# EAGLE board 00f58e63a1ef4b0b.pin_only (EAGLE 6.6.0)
REV: B

Size 55.88 x 22.86 mm. Coordinates in mm from the lower left corner, seen from the top.
Outline: 0,20.32 0,2.54 arc90 2.54,0 53.34,0 arc90 55.88,2.54 55.88,20.32 arc90 53.34,22.86 2.54,22.86 arc90 0,20.32
Copper layers (1*16): Top 0.035mm / dielectric 1.5mm / Bottom 0.035mm
Design rules "adafruit *": minimum track width 8mil, minimum drill 15.5mil, track to track 8mil, track to pad 8mil, pad to pad 8mil, via to via 8mil, smd to smd 8mil, copper to edge 10mil, drill to drill 8mil, minimum pad ring 10mil, minimum via ring 8mil, stop-mask expansion 2mil, vias tented up to drill 20mil, thermal gap 10mil

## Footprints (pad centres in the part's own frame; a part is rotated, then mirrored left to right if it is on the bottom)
0603-NO = smd 1.1 x 1: 1 -0.85,0; 2 0.85,0
0805-NO = smd 1.24 x 1.5: 1 -0.95,0; 2 0.95,0
FIDUCIAL_1MM = smd 1 x 1: 1 0,0
SOT23-5L = smd 0.55 x 1.2: 1 -0.95,-1.3; 2 0,-1.3; 3 0.95,-1.3; 4 0.95,1.3; 5 -0.95,1.3
1X03_ROUND_76 = drill 1 pad 1.93: 1 -2.54,0; 2 0,0; 3 2.54,0
1X13_ROUND_70 = drill 1 pad 1.676: 1 -15.24,0; 2 -12.7,0; 3 -10.16,0; 4 -7.62,0; 5 -5.08,0; 6 -2.54,0; 7 0,0; 8 2.54,0; 9 5.08,0; 10 7.62,0; 11 10.16,0; 12 12.7,0; 13 15.24,0
1X09_ROUND_70 = drill 1 pad 1.778: 1 -10.16,0; 2 -7.62,0; 3 -5.08,0; 4 -2.54,0; 5 0,0; 6 2.54,0; 7 5.08,0; 8 7.62,0; 9 10.16,0
FEATHERWING_NODIM = drill 1 pad 1.778: 1 6.35,1.27; 2 8.89,1.27; 3 11.43,1.27; 4 13.97,1.27; 5 16.51,1.27; 6 19.05,1.27; 7 21.59,1.27; 8 24.13,1.27; 9 26.67,1.27; 10 29.21,1.27; 11 31.75,1.27; 12 34.29,1.27; 13 36.83,1.27; 14 39.37,1.27; 15 41.91,1.27; 16 44.45,1.27; 17 44.45,21.59; 18 41.91,21.59; 19 39.37,21.59; 20 36.83,21.59; 21 34.29,21.59; 22 31.75,21.59; 23 29.21,21.59; 24 26.67,21.59; 25 24.13,21.59; 26 21.59,21.59; 27 19.05,21.59; 28 16.51,21.59 | drill 2.5 pad 3.81: P$1 2.54,20.32; P$2 2.54,2.54 | hole 2.54: 48.26,20.32; 48.26,2.54
SOLDERJUMPER_REFLOW_NOPASTE = smd 1.168 x 1.6: 1 -0.762,0; 2 0.762,0
SOLDERJUMPER_CLOSEDWIRE = smd 1.168 x 1.6: 1 -0.762,0; 2 0.762,0 | smd 0.635 x 0.203: WIRE 0,0
BTN_KMR2_4.6X2.8 = smd 0.9 x 0.9: A 2.05,0.8; A' -2.05,0.8; B 2.05,-0.8; B' -2.05,-0.8
LQFP48 = smd 1.1 x 0.285: 1 -4.2,2.75; 2 -4.2,2.25; 3 -4.2,1.75; 4 -4.2,1.25; 5 -4.2,0.75; 6 -4.2,0.25; 7 -4.2,-0.25; 8 -4.2,-0.75; 9 -4.2,-1.25; 10 -4.2,-1.75; 11 -4.2,-2.25; 12 -4.2,-2.75; 25 4.2,-2.75; 26 4.2,-2.25; 27 4.2,-1.75; 28 4.2,-1.25; 29 4.2,-0.75; 30 4.2,-0.25; 31 4.2,0.25; 32 4.2,0.75; 33 4.2,1.25; 34 4.2,1.75; 35 4.2,2.25; 36 4.2,2.75 | smd 0.285 x 1.1: 13 -2.75,-4.2; 14 -2.25,-4.2; 15 -1.75,-4.2; 16 -1.25,-4.2; 17 -0.75,-4.2; 18 -0.25,-4.2; 19 0.25,-4.2; 20 0.75,-4.2; 21 1.25,-4.2; 22 1.75,-4.2; 23 2.25,-4.2; 24 2.75,-4.2; 37 2.75,4.2; 38 2.25,4.2; 39 1.75,4.2; 40 1.25,4.2; 41 0.75,4.2; 42 0.25,4.2; 43 -0.25,4.2; 44 -0.75,4.2; 45 -1.25,4.2; 46 -1.75,4.2; 47 -2.25,4.2 | smd 0.28 x 1.1: 48 -2.75,4.2
RJ45_PULSEJACK = drill 0.9 pad 1.676: 1 4.445,-6.35; 2 3.175,-8.89; 3 1.905,-6.35; 4 0.635,-8.89; 5 -0.635,-6.35; 6 -1.905,-8.89; 7 -3.175,-6.35; 8 -4.445,-8.89 | drill 1 pad 1.676: 9 6.325,4.9; 10 3.785,3.38; 11 -3.785,4.9; 12 -6.325,3.38 | drill 1.6: P$5 -7.875,-3.05; P$6 7.875,-3.05 | hole 3.2: -5.715,0; 5.715,0
CRYSTAL_3.2X2.5 = smd 1.4 x 1.2: 1 -1.1,-0.8; 2 1.1,0.8; GND1 -1.1,0.8; GND2 1.1,-0.8

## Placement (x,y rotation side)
C1  22pF  [0603-NO]  7.62,8.64 180 top
C2  22pF  [0603-NO]  7.24,14.48 180 top
C3  6.8nF  [0603-NO]  35.56,15.88 180 top
C4  6.8nF  [0603-NO]  35.56,17.27 180 top
C5  10nF  [0603-NO]  35.56,13.08 180 top
C6  10nF  [0603-NO]  35.56,10.29 180 top
C7  0.1uF  [0603-NO]  22.73,16.13 270 top
C8  0.1uF  [0603-NO]  24.13,16.13 270 top
C9  0.1uF  [0603-NO]  25.53,16.13 270 top
C10  0.1uF  [0603-NO]  26.92,16.13 270 top
C11  10uF  [0805-NO]  28.57,16.13 270 top
C12  10uF  [0805-NO]  13.97,20.07 90 top
C13  0.1uF  [0603-NO]  12.83,16.76 180 top
C14  10uF  [0805-NO]  6.6,6.22 90 top
C15  0.1uF  [0603-NO]  8.38,6.35 90 top
FB1  ferrite  [0805-NO]  10.79,18.29 0 top
FB2  ferrite  [0805-NO]  29.08,7.87 0 top
FID1  FIDUCIAL""  [FIDUCIAL_1MM]  46.48,1.02 0 top
FID2  FIDUCIAL""  [FIDUCIAL_1MM]  1.02,5.21 0 top
FID3  FIDUCIAL""  [FIDUCIAL_1MM]  46.48,21.84 0 top
IC1  74AHC1G125  [SOT23-5L]  11.05,7.37 180 top
JP1  [1X03_ROUND_76]  2.54,11.43 270 top
JP2  [1X13_ROUND_70]  21.59,3.3 180 top
JP4  [1X09_ROUND_70]  26.67,19.43 0 top
MS1  FEATHERWING_NODIM  [FEATHERWING_NODIM]  0,0 0 top
R1  12.4K  [0603-NO]  24.51,13.59 0 top
R2  1M  [0603-NO]  10.16,11.18 90 top
R3  10K  [0603-NO]  3.94,17.14 0 top
R4  49.9  [0603-NO]  35.56,7.49 180 top
R5  10K  [0603-NO]  25.65,8.13 180 top
R6  10K  [0603-NO]  25.65,6.73 180 top
R7  10K  [0603-NO]  25.65,5.4 180 top
R8  10K  [0603-NO]  13.74,6.48 90 top
R9  49.9  [0603-NO]  35.56,6.1 180 top
R10  49.9  [0603-NO]  35.56,14.48 180 top
R11  49.9  [0603-NO]  35.56,11.68 180 top
R12  10  [0603-NO]  35.56,8.89 180 top
R13  470  [0603-NO]  53.21,20.83 180 top
R14  470  [0603-NO]  53.21,2.16 180 top
R15  10K  [0603-NO]  3.94,15.75 0 top
SJ1  [SOLDERJUMPER_REFLOW_NOPASTE]  18.29,11.68 0 bottom
SJ2  [SOLDERJUMPER_REFLOW_NOPASTE]  18.29,9.4 0 bottom
SJ3  [SOLDERJUMPER_REFLOW_NOPASTE]  18.29,7.11 180 bottom
SJ4  [SOLDERJUMPER_CLOSEDWIRE]  5.84,17.53 180 bottom
SW1  KMR2  [BTN_KMR2_4.6X2.8]  7.75,20.95 180 top
U$1  W5500  [LQFP48]  17.78,11.43 180 top
U$45  [PCBFEAT-REV-040]  27.69,12.7 0 top
U$48  [FEATHERLOGO_MED]  39.24,8.38 0 bottom
U$49  [ADAFRUIT_3.5MM]  30.1,13.21 0 top
X1  RB1-125BAG1A  [RJ45_PULSEJACK]  48.77,11.43 270 top
Y1  25MHz  [CRYSTAL_3.2X2.5]  7.62,11.43 90 top

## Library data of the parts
C1-C15 FB1 FB2 JP1 JP2 JP4 MS1 R1-R15 SJ1-SJ4 SW1 U$1 U$45 U$48 U$49 X1 Y1 = microbuilder
FID1-FID3 = microbuilder; BOM: EXCLUDE
IC1 = adafruit

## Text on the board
tPlace: 4 x Not Plated Holes | Act | Reset | CS | IRQ | Ethernet / FeatherWing | RST | Link
bPlace: CS | VBAT | EN | USB | CS | Uses SPI / & CS Pin | WIZnet W5500 / Ethernet / Feather / Wing | M0 | M1 | M2 | MODE | RST | 3V | GND | SCK | MOSI | MISO

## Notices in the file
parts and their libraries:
microbuilder: This work is placed in the public domain, and may be freely used for commercial and non-commercial work with the following conditions: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
